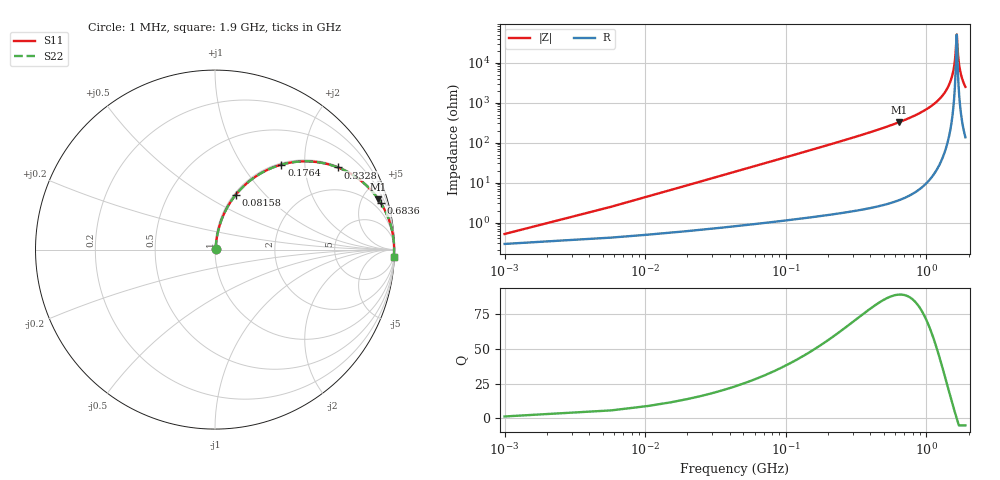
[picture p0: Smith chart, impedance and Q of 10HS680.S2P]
! Coilcraft 1008HS-680 Chip Inductor
! 02 July 2002
# MHZ S MA R 50
!Freq  MagS11  AngS11  MagS21  AngS21  MagS12  AngS12  MagS22  AngS22
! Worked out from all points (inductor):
!   402 points, 1 MHz to 1.9 GHz, reference 50 ohm
!   read as one part in series: L = 68 nH near 10.48 MHz
!   highest Q = 89.1 at 640.9 MHz (marker M1), where L = 80.1 nH
!   self-resonance near 1.646 GHz
!   S11 on the Smith chart (normalised r, x): 1 MHz: 1.01, +0.01; 81.58 MHz: 1.02, +0.70; 176.4 MHz: 1.03, +1.52; 332.8 MHz: 1.04, +2.96; 683.6 MHz: 1.08, +7.05; 1.9 GHz: 4, -49
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1  0.00516 55.4  0.9971 -0.2  0.9971 -0.2  0.00516 55.4
15.22  0.06478 81.4  0.9924 -3.7  0.9924 -3.7  0.06478 81.4
24.7  0.1045 80.4  0.9881 -6.0  0.9881 -6.0  0.1045 80.4
48.4  0.2012 76.1  0.9714 -11.6  0.9714 -11.6  0.2012 76.1
81.58  0.327 69.2  0.9354 -19.1  0.9354 -19.1  0.327 69.2
176.38  0.6008 52.0  0.788 -36.9  0.788 -36.9  0.6008 52.0
318.58  0.8111 35.0  0.5736 -54.2  0.5736 -54.2  0.8111 35.0
332.8  0.8238 33.8  0.5557 -55.5  0.5557 -55.5  0.8238 33.8
636.16  0.9513 17.3  0.2979 -72.0  0.2979 -72.0  0.9513 17.3
640.9  0.9521 17.2  0.2952 -72.2  0.2952 -72.2  0.9521 17.2
683.56  0.9592 15.8  0.272 -73.6  0.272 -73.6  0.9592 15.8
953.74  0.9848 9.3  0.1608 -80.0  0.1608 -80.0  0.9848 9.3
1271.32  0.9954 4.3  0.07434 -84.3  0.07434 -84.3  0.9954 4.3
1470.4  0.9976 1.9  0.03258 -84.9  0.03258 -84.9  0.9976 1.9
1584.16  0.998 0.7  0.01152 -79.8  0.01152 -79.8  0.998 0.7
1607.86  0.998 0.4  0.007409 -74.5  0.007409 -74.5  0.998 0.4
1641.04  0.998 0.1  0.002383 -34.9  0.002383 -34.9  0.998 0.1
1650.52  0.998 -0.0  0.001977 7.7  0.001977 7.7  0.998 -0.0
1688.44  0.998 -0.4  0.006989 73.1  0.006989 73.1  0.998 -0.4
1731.1  0.9979 -0.8  0.01392 80.8  0.01392 80.8  0.9979 -0.8
1802.2  0.9976 -1.4  0.02528 83.8  0.02528 83.8  0.9976 -1.4
1900  0.997 -2.3  0.04029 84.6  0.04029 84.6  0.997 -2.3
